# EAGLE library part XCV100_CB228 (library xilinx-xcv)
xcv100_cb228_1532 edit this description Auto generated by make-symbol-device-package-bsdl.ulp Rev. 26 Source: xcv100_cb228_1532.bsd
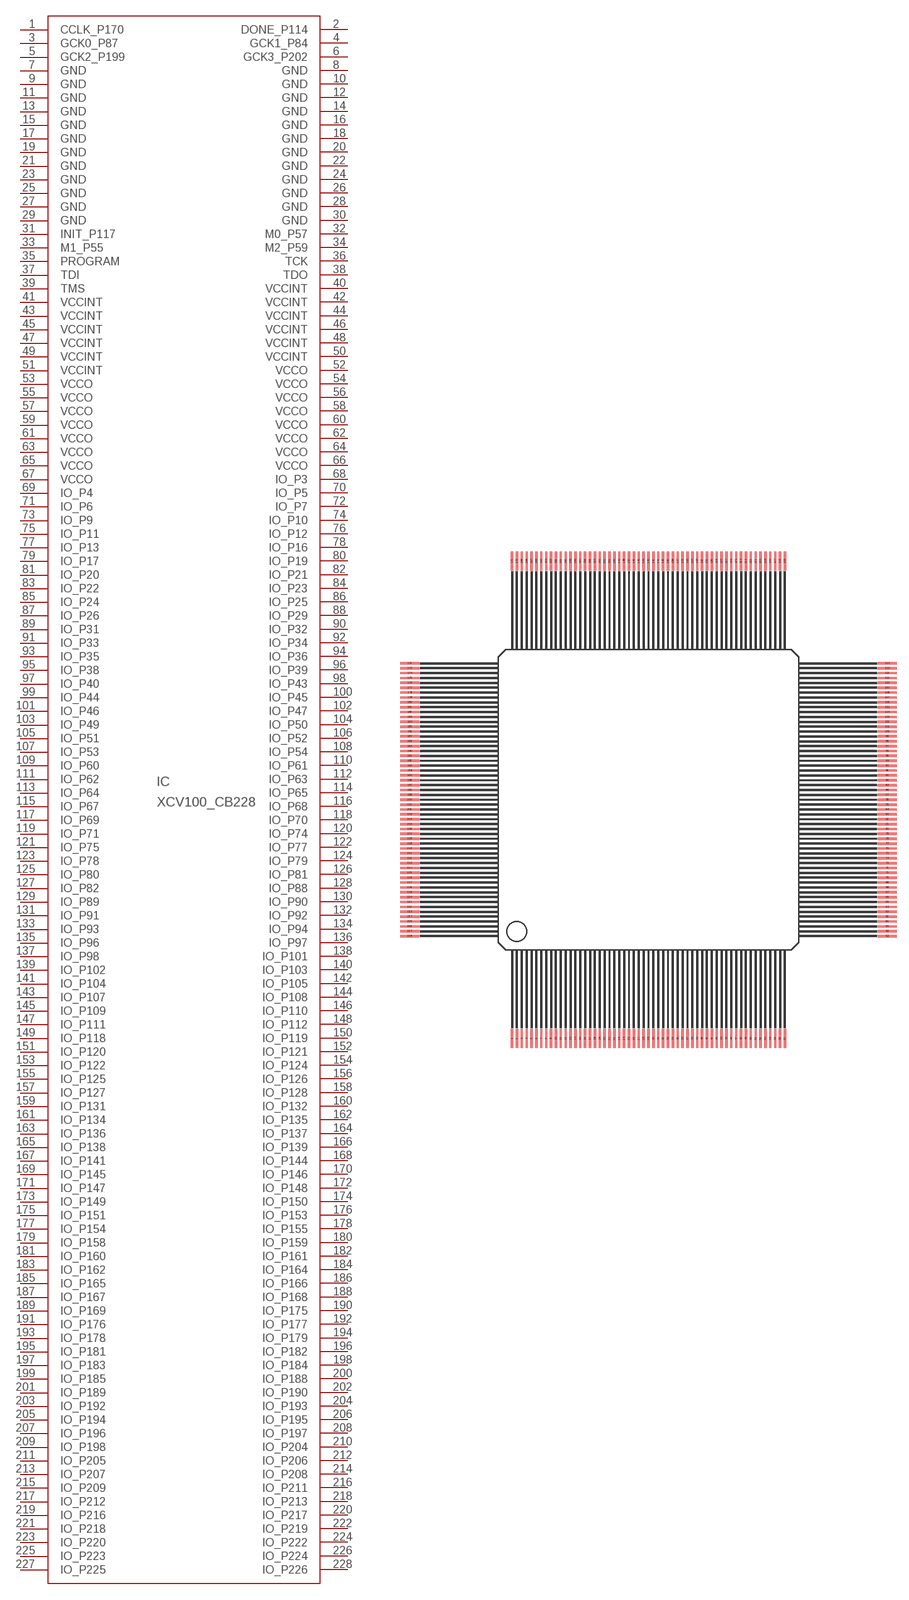
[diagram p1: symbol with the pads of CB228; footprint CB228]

Designator prefix IC

## XCV100_CB228 (OC_FARNELL: unknown; OC_NEWARK: unknown)  [CB228]
1  CCLK_P170
2  DONE_P114
3  GCK0_P87  in
4  GCK1_P84  in
5  GCK2_P199  in
6  GCK3_P202  in
7  GND  pwr
8  GND  pwr
9  GND  pwr
10  GND  pwr
11  GND  pwr
12  GND  pwr
13  GND  pwr
14  GND  pwr
15  GND  pwr
16  GND  pwr
17  GND  pwr
18  GND  pwr
19  GND  pwr
20  GND  pwr
21  GND  pwr
22  GND  pwr
23  GND  pwr
24  GND  pwr
25  GND  pwr
26  GND  pwr
27  GND  pwr
28  GND  pwr
29  GND  pwr
30  GND  pwr
31  INIT_P117
32  M0_P57  in
33  M1_P55  in
34  M2_P59  in
35  PROGRAM  in
36  TCK  in
37  TDI  in
38  TDO  out
39  TMS  in
40  VCCINT  pwr
41  VCCINT  pwr
42  VCCINT  pwr
43  VCCINT  pwr
44  VCCINT  pwr
45  VCCINT  pwr
46  VCCINT  pwr
47  VCCINT  pwr
48  VCCINT  pwr
49  VCCINT  pwr
50  VCCINT  pwr
51  VCCINT  pwr
52  VCCO  pwr
53  VCCO  pwr
54  VCCO  pwr
55  VCCO  pwr
56  VCCO  pwr
57  VCCO  pwr
58  VCCO  pwr
59  VCCO  pwr
60  VCCO  pwr
61  VCCO  pwr
62  VCCO  pwr
63  VCCO  pwr
64  VCCO  pwr
65  VCCO  pwr
66  VCCO  pwr
67  VCCO  pwr
68  IO_P3
69  IO_P4
70  IO_P5
71  IO_P6
72  IO_P7
73  IO_P9
74  IO_P10
75  IO_P11
76  IO_P12
77  IO_P13
78  IO_P16
79  IO_P17
80  IO_P19
81  IO_P20
82  IO_P21
83  IO_P22
84  IO_P23
85  IO_P24
86  IO_P25
87  IO_P26
88  IO_P29
89  IO_P31
90  IO_P32
91  IO_P33
92  IO_P34
93  IO_P35
94  IO_P36
95  IO_P38
96  IO_P39
97  IO_P40
98  IO_P43
99  IO_P44
100  IO_P45
101  IO_P46
102  IO_P47
103  IO_P49
104  IO_P50
105  IO_P51
106  IO_P52
107  IO_P53
108  IO_P54
109  IO_P60
110  IO_P61
111  IO_P62
112  IO_P63
113  IO_P64
114  IO_P65
115  IO_P67
116  IO_P68
117  IO_P69
118  IO_P70
119  IO_P71
120  IO_P74
121  IO_P75
122  IO_P77
123  IO_P78
124  IO_P79
125  IO_P80
126  IO_P81
127  IO_P82
128  IO_P88
129  IO_P89
130  IO_P90
131  IO_P91
132  IO_P92
133  IO_P93
134  IO_P94
135  IO_P96
136  IO_P97
137  IO_P98
138  IO_P101
139  IO_P102
140  IO_P103
141  IO_P104
142  IO_P105
143  IO_P107
144  IO_P108
145  IO_P109
146  IO_P110
147  IO_P111
148  IO_P112
149  IO_P118
150  IO_P119
151  IO_P120
152  IO_P121
153  IO_P122
154  IO_P124
155  IO_P125
156  IO_P126
157  IO_P127
158  IO_P128
159  IO_P131
160  IO_P132
161  IO_P134
162  IO_P135
163  IO_P136
164  IO_P137
165  IO_P138
166  IO_P139
167  IO_P141
168  IO_P144
169  IO_P145
170  IO_P146
171  IO_P147
172  IO_P148
173  IO_P149
174  IO_P150
175  IO_P151
176  IO_P153
177  IO_P154
178  IO_P155
179  IO_P158
180  IO_P159
181  IO_P160
182  IO_P161
183  IO_P162
184  IO_P164
185  IO_P165
186  IO_P166
187  IO_P167
188  IO_P168
189  IO_P169
190  IO_P175
191  IO_P176
192  IO_P177
193  IO_P178
194  IO_P179
195  IO_P181
196  IO_P182
197  IO_P183
198  IO_P184
199  IO_P185
200  IO_P188
201  IO_P189
202  IO_P190
203  IO_P192
204  IO_P193
205  IO_P194
206  IO_P195
207  IO_P196
208  IO_P197
209  IO_P198
210  IO_P204
211  IO_P205
212  IO_P206
213  IO_P207
214  IO_P208
215  IO_P209
216  IO_P211
217  IO_P212
218  IO_P213
219  IO_P216
220  IO_P217
221  IO_P218
222  IO_P219
223  IO_P220
224  IO_P222
225  IO_P223
226  IO_P224
227  IO_P225
228  IO_P226

## Footprint CB228 (pad centres in mm)
Ceramic Brazed CQFP (CB228) Package Source: cb228.pdf
smd 0.305 x 2.54: 1 -17.78,-31.115; 2 -17.145,-31.115; 3 -16.51,-31.115; 4 -15.875,-31.115; 5 -15.24,-31.115; 6 -14.605,-31.115; 7 -13.97,-31.115; 8 -13.335,-31.115; 9 -12.7,-31.115; 10 -12.065,-31.115; 11 -11.43,-31.115; 12 -10.795,-31.115; 13 -10.16,-31.115; 14 -9.525,-31.115; 15 -8.89,-31.115; 16 -8.255,-31.115; 17 -7.62,-31.115; 18 -6.985,-31.115; 19 -6.35,-31.115; 20 -5.715,-31.115; 21 -5.08,-31.115; 22 -4.445,-31.115; 23 -3.81,-31.115; 24 -3.175,-31.115; 25 -2.54,-31.115; 26 -1.905,-31.115; 27 -1.27,-31.115; 28 -0.635,-31.115; 29 0,-31.115; 30 0.635,-31.115; 31 1.27,-31.115; 32 1.905,-31.115; 33 2.54,-31.115; 34 3.175,-31.115; 35 3.81,-31.115; 36 4.445,-31.115; 37 5.08,-31.115; 38 5.715,-31.115; 39 6.35,-31.115; 40 6.985,-31.115; 41 7.62,-31.115; 42 8.255,-31.115; 43 8.89,-31.115; 44 9.525,-31.115; 45 10.16,-31.115; 46 10.795,-31.115; 47 11.43,-31.115; 48 12.065,-31.115; 49 12.7,-31.115; 50 13.335,-31.115; 51 13.97,-31.115; 52 14.605,-31.115; 53 15.24,-31.115; 54 15.875,-31.115; 55 16.51,-31.115; 56 17.145,-31.115; 57 17.78,-31.115; 115 17.78,31.115; 116 17.145,31.115; 117 16.51,31.115; 118 15.875,31.115; 119 15.24,31.115; 120 14.605,31.115; 121 13.97,31.115; 122 13.335,31.115; 123 12.7,31.115; 124 12.065,31.115; 125 11.43,31.115; 126 10.795,31.115; 127 10.16,31.115; 128 9.525,31.115; 129 8.89,31.115; 130 8.255,31.115; 131 7.62,31.115; 132 6.985,31.115; 133 6.35,31.115; 134 5.715,31.115; 135 5.08,31.115; 136 4.445,31.115; 137 3.81,31.115; 138 3.175,31.115; 139 2.54,31.115; 140 1.905,31.115; 141 1.27,31.115; 142 0.635,31.115; 143 0,31.115; 144 -0.635,31.115; 145 -1.27,31.115; 146 -1.905,31.115; 147 -2.54,31.115; 148 -3.175,31.115; 149 -3.81,31.115; 150 -4.445,31.115; 151 -5.08,31.115; 152 -5.715,31.115; 153 -6.35,31.115; 154 -6.985,31.115; 155 -7.62,31.115; 156 -8.255,31.115; 157 -8.89,31.115; 158 -9.525,31.115; 159 -10.16,31.115; 160 -10.795,31.115; 161 -11.43,31.115; 162 -12.065,31.115; 163 -12.7,31.115; 164 -13.335,31.115; 165 -13.97,31.115; 166 -14.605,31.115; 167 -15.24,31.115; 168 -15.875,31.115; 169 -16.51,31.115; 170 -17.145,31.115; 171 -17.78,31.115
smd 2.54 x 0.305: 58 31.115,-17.78; 59 31.115,-17.145; 60 31.115,-16.51; 61 31.115,-15.875; 62 31.115,-15.24; 63 31.115,-14.605; 64 31.115,-13.97; 65 31.115,-13.335; 66 31.115,-12.7; 67 31.115,-12.065; 68 31.115,-11.43; 69 31.115,-10.795; 70 31.115,-10.16; 71 31.115,-9.525; 72 31.115,-8.89; 73 31.115,-8.255; 74 31.115,-7.62; 75 31.115,-6.985; 76 31.115,-6.35; 77 31.115,-5.715; 78 31.115,-5.08; 79 31.115,-4.445; 80 31.115,-3.81; 81 31.115,-3.175; 82 31.115,-2.54; 83 31.115,-1.905; 84 31.115,-1.27; 85 31.115,-0.635; 86 31.115,0; 87 31.115,0.635; 88 31.115,1.27; 89 31.115,1.905; 90 31.115,2.54; 91 31.115,3.175; 92 31.115,3.81; 93 31.115,4.445; 94 31.115,5.08; 95 31.115,5.715; 96 31.115,6.35; 97 31.115,6.985; 98 31.115,7.62; 99 31.115,8.255; 100 31.115,8.89; 101 31.115,9.525; 102 31.115,10.16; 103 31.115,10.795; 104 31.115,11.43; 105 31.115,12.065; 106 31.115,12.7; 107 31.115,13.335; 108 31.115,13.97; 109 31.115,14.605; 110 31.115,15.24; 111 31.115,15.875; 112 31.115,16.51; 113 31.115,17.145; 114 31.115,17.78; 172 -31.115,17.78; 173 -31.115,17.145; 174 -31.115,16.51; 175 -31.115,15.875; 176 -31.115,15.24; 177 -31.115,14.605; 178 -31.115,13.97; 179 -31.115,13.335; 180 -31.115,12.7; 181 -31.115,12.065; 182 -31.115,11.43; 183 -31.115,10.795; 184 -31.115,10.16; 185 -31.115,9.525; 186 -31.115,8.89; 187 -31.115,8.255; 188 -31.115,7.62; 189 -31.115,6.985; 190 -31.115,6.35; 191 -31.115,5.715; 192 -31.115,5.08; 193 -31.115,4.445; 194 -31.115,3.81; 195 -31.115,3.175; 196 -31.115,2.54; 197 -31.115,1.905; 198 -31.115,1.27; 199 -31.115,0.635; 200 -31.115,0; 201 -31.115,-0.635; 202 -31.115,-1.27; 203 -31.115,-1.905; 204 -31.115,-2.54; 205 -31.115,-3.175; 206 -31.115,-3.81; 207 -31.115,-4.445; 208 -31.115,-5.08; 209 -31.115,-5.715; 210 -31.115,-6.35; 211 -31.115,-6.985; 212 -31.115,-7.62; 213 -31.115,-8.255; 214 -31.115,-8.89; 215 -31.115,-9.525; 216 -31.115,-10.16; 217 -31.115,-10.795; 218 -31.115,-11.43; 219 -31.115,-12.065; 220 -31.115,-12.7; 221 -31.115,-13.335; 222 -31.115,-13.97; 223 -31.115,-14.605; 224 -31.115,-15.24; 225 -31.115,-15.875; 226 -31.115,-16.51; 227 -31.115,-17.145; 228 -31.115,-17.78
